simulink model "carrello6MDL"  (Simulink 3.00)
settings: Solver=ode45  SolverMode=SingleTasking  StartTime=0.0  StopTime=10.0  RelTol=1e-6  AbsTol=1e-7
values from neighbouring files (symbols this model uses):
  Am = [-b1/Ma -K/Ma       b1/Ma      0 0    [carrello2.M]    (also in carrello3.M; carrello4.M; carrello5.M; carrello6.M)
  B1 = Bm(:,1)    [carrello4.M]    (also in carrello5.M; carrello6.M)
  b1 = 2*1500*N/(m/sec)    (= 3000)    [carrello2.M]    (also in carrello3.M; carrello4.M; carrello5.M; carrello6.M)
  b2 = 2*1500*N/(m/sec)    (= 3000)    [carrello2.M]    (also in carrello3.M; carrello4.M; carrello5.M; carrello6.M)
  C1 = Cm(1,:)    [carrello4.M]    (also in carrello5.M; carrello6.M; carrello1.M = [1 0 0 0 0])
  K = 0.8*1800*N/cm    (= 144000)    [carrello2.M]    (also in carrello3.M; carrello4.M; carrello5.M; carrello6.M)
  KK = [KK 0]    [carrello5.M]    (also in carrello6.M)
  Kp = 2*1800*N/cm    (= 360000)    [carrello2.M]    (also in carrello3.M; carrello4.M; carrello5.M; carrello6.M)
  Kr = 1    [carrello5.M]    (also in carrello6.M)
  L = L'    [carrello6.M]
  Ma = 3850*Kg    (= 3850)    [carrello2.M]    (also in carrello3.M; carrello4.M; carrello5.M; carrello6.M)
  mr = 2*134*Kg+524*Kg    (= 792)    [carrello2.M]    (also in carrello3.M; carrello4.M; carrello5.M; carrello6.M)
  R = 1    [carrello4.M]    (also in carrello5.M = 0.1; carrello6.M = 0.1)
  X_0_oss = [0.000000001 0 0 0 0]    [carrello6.M]
  X_12_0 = -Mag/K    (= -0.26228125)    [carrello2.M]    (also in carrello3.M = 0; carrello4.M = 0; carrello5.M = 0; carrello6.M = 0)
  X_20_0 = -(Mag+mrg)/Kp    (= -0.1264945)    [carrello2.M]    (also in carrello3.M = 0; carrello4.M = 0; carrello5.M = 0; carrello6.M = 0)
  Xsdot = 0    [carrello3.M]    (also in carrello4.M; carrello5.M; carrello6.M)
libraries: simulink3 x5

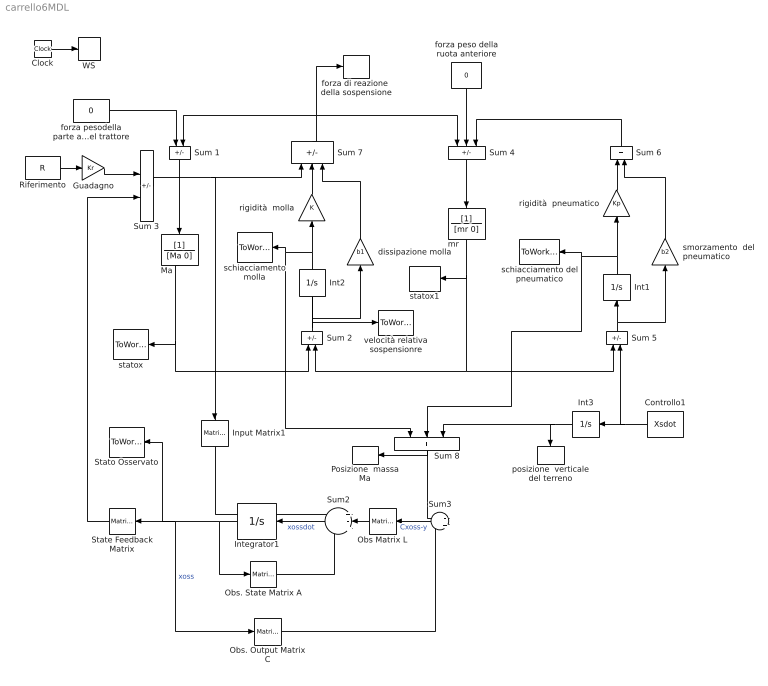
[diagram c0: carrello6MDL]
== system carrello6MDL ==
  Clock : Clock
  Controllo1 : Constant  Orientation=left  Value=Xsdot
  Guadagno : Gain  Gain=Kr  SaturateOnIntegerOverflow=on
  Input Matrix1 : simulink3/Math/Matrix Gain  Orientation=down  K=B1
  Int1 : Integrator  Orientation=up  ExternalReset=none  InitialConditionSource=internal  InitialCondition=X_20_0  LimitOutput=off  UpperSaturationLimit=inf  LowerSaturationLimit=-inf  ShowSaturationPort=off  ShowStatePort=off  AbsoluteTolerance=auto
  Int2 : Integrator  Orientation=up  ExternalReset=none  InitialConditionSource=internal  InitialCondition=X_12_0  LimitOutput=off  UpperSaturationLimit=inf  LowerSaturationLimit=-inf  ShowSaturationPort=off  ShowStatePort=off  AbsoluteTolerance=auto
  Int3 : Integrator  Orientation=left  ExternalReset=none  InitialConditionSource=internal  InitialCondition=X_20_0  LimitOutput=off  UpperSaturationLimit=inf  LowerSaturationLimit=-inf  ShowSaturationPort=off  ShowStatePort=off  AbsoluteTolerance=auto
  Integrator1 : Integrator  Orientation=left  ExternalReset=none  InitialConditionSource=internal  InitialCondition=X_0_oss  LimitOutput=off  UpperSaturationLimit=inf  LowerSaturationLimit=-inf  ShowSaturationPort=off  ShowStatePort=off  AbsoluteTolerance=auto
  Ma : TransferFcn  Orientation=down  Numerator=[1]  Denominator=[Ma 0]
  Obs Matrix L : simulink3/Math/Matrix Gain  Orientation=left  K=L
  Obs. Output Matrix C : simulink3/Math/Matrix Gain  K=C1
  Obs. State Matrix A : simulink3/Math/Matrix Gain  K=Am
  Posizione  massa Ma : ToWorkspace  VariableName=X_Ma  SampleTime=-1  SaveFormat=Matrix
  Riferimento : Constant  Value=R
  State Feedback Matrix : simulink3/Math/Matrix Gain  Orientation=left  K=KK
  Stato Osservato : ToWorkspace  VariableName=Xoss  SampleTime=-1  SaveFormat=Matrix
  Sum 1 : Sum  Orientation=down  Inputs=+-  SaturateOnIntegerOverflow=on
  Sum 2 : Sum  Orientation=up  Inputs=+-
  Sum 3 : Sum  Inputs=+-
  Sum 4 : Sum  Orientation=down  Inputs=++-
  Sum 5 : Sum  Orientation=up  Inputs=+-
  Sum 6 : Sum  Orientation=up  Inputs=++
  Sum 7 : Sum  Orientation=up  Inputs=-++
  Sum 8 : Sum  Orientation=down  Inputs=+++
  Sum2 : Sum  Orientation=left  Inputs=+-+  SaturateOnIntegerOverflow=on
  Sum3 : Sum  Orientation=left  Inputs=-|+  SaturateOnIntegerOverflow=on
  WS : ToWorkspace  VariableName=t  SampleTime=-1  SaveFormat=Matrix
  dissipazione molla : Gain  Orientation=up  Gain=b1  SaturateOnIntegerOverflow=on
  forza di reazione  della sospensione : ToWorkspace  VariableName=R  SampleTime=-1  SaveFormat=Matrix
  forza peso della ruota anteriore : Constant  Orientation=down  Value=0
  forza pesodella parte anteriore del trattore : Constant  Value=0
  mr : TransferFcn  Orientation=down  Numerator=[1]  Denominator=[mr 0]
  posizione  verticale del terreno : ToWorkspace  VariableName=Xs  SampleTime=-1  SaveFormat=Matrix
  rigidità  molla : Gain  Orientation=up  Gain=K  SaturateOnIntegerOverflow=on
  rigidità  pneumatico : Gain  Orientation=up  Gain=Kp  SaturateOnIntegerOverflow=on
  schiacciamento del pneumatico : ToWorkspace  VariableName=X_20  SampleTime=-1  SaveFormat=Matrix
  schiacciamento molla : ToWorkspace  VariableName=X_12  SampleTime=-1  SaveFormat=Matrix
  smorzamento  del pneumatico : Gain  Orientation=up  Gain=b2  SaturateOnIntegerOverflow=on
  statox : ToWorkspace  VariableName=x1  SampleTime=-1  SaveFormat=Matrix
  statox1 : ToWorkspace  VariableName=x3  SampleTime=-1  SaveFormat=Matrix
  velocità relativa sospensionre : ToWorkspace  VariableName=vel_rel  SampleTime=-1  SaveFormat=Matrix
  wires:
  forza pesodella parte anteriore del trattore/1 -> Sum 1/1
  Sum 1/1 -> Ma/1
  forza peso della ruota anteriore/1 -> Sum 4/2
  Sum 4/1 -> mr/1
  Int1/1 -> rigidità  pneumatico/1, schiacciamento del pneumatico/1, Sum 8/2
  Sum 5/1 -> Int1/1, smorzamento  del pneumatico/1
  rigidità  pneumatico/1 -> Sum 6/1
  smorzamento  del pneumatico/1 -> Sum 6/2
  Sum 7/1 -> Sum 1/2, forza di reazione  della sospensione/1, Sum 4/1
  Sum 6/1 -> Sum 4/3
  Sum 2/1 -> velocità relativa sospensionre/1, Int2/1, dissipazione molla/1
  Int2/1 -> rigidità  molla/1, schiacciamento molla/1, Sum 8/1
  dissipazione molla/1 -> Sum 7/3
  rigidità  molla/1 -> Sum 7/2
  Controllo1/1 -> Int3/1, Sum 5/2
  Int3/1 -> Sum 8/3, posizione  verticale del terreno/1
  Clock/1 -> WS/1
  Riferimento/1 -> Guadagno/1
  Guadagno/1 -> Sum 3/1
  Integrator1/1 -> Obs. State Matrix A/1, Obs. Output Matrix C/1, State Feedback Matrix/1, Stato Osservato/1  "xoss"
  Sum2/1 -> Integrator1/1  "xossdot"
  Obs. State Matrix A/1 -> Sum2/3
  Obs. Output Matrix C/1 -> Sum3/2
  Obs Matrix L/1 -> Sum2/2
  Sum3/1 -> Obs Matrix L/1  "Cxoss-y"
  Sum 8/1 -> Posizione  massa Ma/1, Sum3/1
  Input Matrix1/1 -> Sum2/1
  Sum 3/1 -> Sum 7/1, Input Matrix1/1
  State Feedback Matrix/1 -> Sum 3/2
  Ma/1 -> Sum 2/1, statox/1
  mr/1 -> Sum 5/1, Sum 2/2, statox1/1
